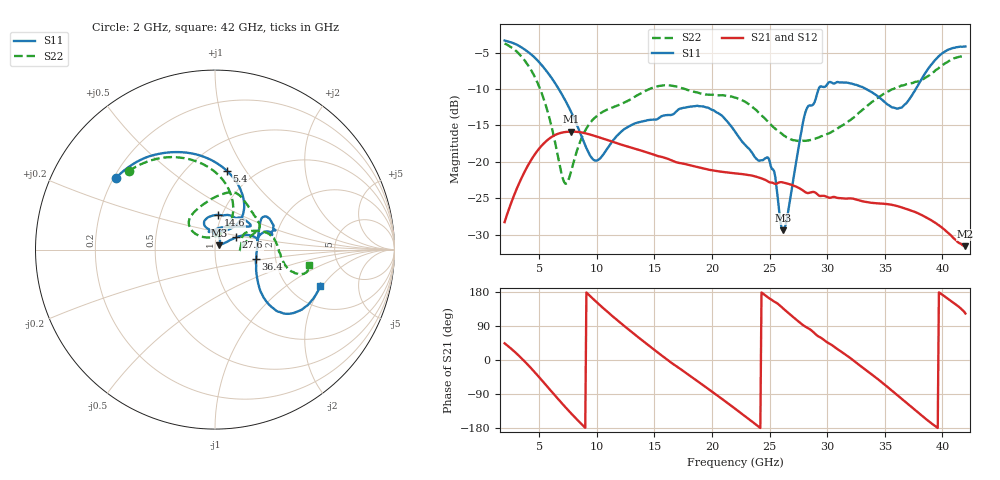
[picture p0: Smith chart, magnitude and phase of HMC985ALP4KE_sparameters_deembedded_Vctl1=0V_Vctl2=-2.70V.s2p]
!s2p File: Measurements: S11, S21, S12, S22
# GHz S dB R 50.0
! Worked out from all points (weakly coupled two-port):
!   401 points, 2 GHz to 42 GHz, reference 50 ohm
!   highest |S21| = -15.84 dB at 7.8 GHz (marker M1); lowest = -31.6 dB at 42 GHz (marker M2)
!   lowest |S11| = -29.4 dB at 26.2 GHz (marker M3), VSWR 1.07, Z = 52.3 + j2.61 ohm
!   |S11| at or under -10 dB: 6.701 GHz to 29.26 GHz (22.56 GHz wide, 125 % of centre); 33.38 GHz to 37.7 GHz (4.315 GHz wide, 12.1 % of centre)
!   |S22| runs from -23.0 to -3.7 dB; largest |S21 - S12| = 0.00063
!   S11 on the Smith chart (normalised r, x): 2 GHz: 0.21, +0.31; 5.4 GHz: 0.75, +0.82; 14.6 GHz: 0.96, +0.39; 27.6 GHz: 1.26, +0.17; 36.4 GHz: 1.58, -0.18; 42 GHz: 2.91, -1.90
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2  -3.33 144.2  -28.28 44.0  -28.26 44.0  -3.75 137.7
3.5  -4.32 117.7  -22.12 3.6  -22.14 3.6  -5.61 106.1
5.4  -7.06 81.4  -17.47 -59.4  -17.49 -59.4  -11.38 68.1
7.1  -11.08 54.5  -15.94 -118.6  -15.96 -118.6  -22.50 85.8
7.8  -13.23 49.4  -15.84 -141.7  -15.84 -141.7  -21.13 128.9
8.7  -16.58 52.7  -15.97 -169.9  -15.97 -169.9  -16.66 141.3
10  -19.82 87.9  -16.52 152.3  -16.51 152.3  -13.69 135.0
14.6  -14.23 84.5  -18.82 36.0  -18.79 36.0  -9.98 80.6
15.4  -13.97 73.8  -19.24 17.5  -19.27 17.4  -9.58 74.2
19.3  -12.40 33.9  -20.92 -68.0  -20.94 -68.0  -10.66 43.5
22  -15.83 52.2  -21.57 -128.3  -21.59 -128.3  -11.17 26.3
25  -19.88 99.2  -22.81 162.4  -22.79 162.4  -14.71 15.3
26.2  -29.41 47.3  -22.84 135.5  -22.87 135.4  -16.32 4.7
27.6  -17.28 29.9  -23.63 99.4  -23.66 99.3  -17.09 -1.6
28.1  -13.26 21.0  -24.16 88.2  -24.20 88.2  -17.11 -0.3
28.7  -12.23 13.1  -24.14 76.4  -24.12 76.4  -16.91 3.6
31  -9.05 23.3  -24.97 26.6  -24.95 26.6  -15.30 26.2
33.3  -9.93 34.1  -25.48 -24.7  -25.48 -24.8  -12.57 26.2
35.4  -12.27 11.9  -25.84 -75.3  -25.83 -75.3  -10.26 17.2
36.4  -12.58 -13.2  -26.21 -100.8  -26.24 -100.8  -9.55 11.2
39.5  -5.82 -43.4  -28.48 -177.2  -28.47 -177.1  -7.32 -14.9
42  -4.15 -18.9  -31.57 122.7  -31.56 122.8  -5.50 -9.6
